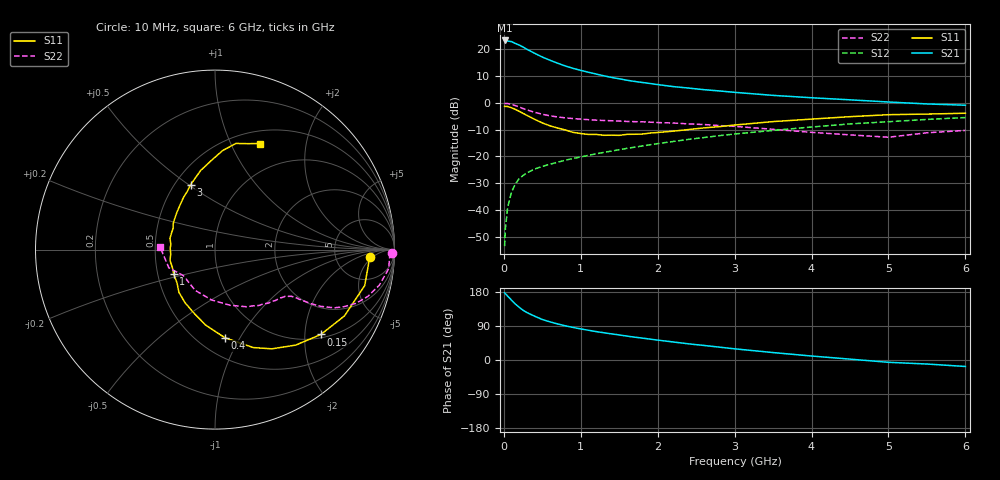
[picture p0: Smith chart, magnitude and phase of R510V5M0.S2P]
! SIEMENS Small Signal Semiconductors
! BFR183
! Si NPN RF Bipolar Junction Transistor in SOT23
! VCE = 10 V  IC = 5 mA
! Common Emitter S-Parameters:  May  1996
# GHz  S  MA  R  50
!  f  S11  S21  S12  S22
! GHz  MAG  ANG  MAG  ANG  MAG  ANG  MAG  ANG
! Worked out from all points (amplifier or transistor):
!   36 points, 10 MHz to 6 GHz, reference 50 ohm
!   highest |S21| = 23.4 dB at 10 MHz (marker M1)
!   |S21| within 3 dB of that: start of sweep to 282.1 MHz
!   unconditionally stable (mu >= 1): 1.095 GHz to 2.758 GHz
!   at 250 MHz: K = 0.41, MSG = 24.0 dB, |S12| = -27.1 dB
!   at 1.4 GHz: K = 1.05, MAG = 12.4 dB, |S12| = -18.0 dB
!   at 6 GHz: K = 0.87, MSG = 2.3 dB, |S12| = -5.5 dB
!   S11 on the Smith chart (normalised r, x): 10 MHz: 12, -4; 150 MHz: 1.09, -2.41; 400 MHz: 0.67, -0.87; 1 GHz: 0.61, -0.18; 3 GHz: 0.60, +0.51; 6 GHz: 0.64, +1.30
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0.01  0.8619 -2.9  14.71 177.5  0.0021 87.9  0.985 -1.2
0.02  0.8593 -5.3  14.47 174.9  0.0045 85.7  0.9738 -2.6
0.05  0.8579 -13.5  14.38 168.6  0.0112 81.7  0.9735 -6.3
0.1  0.8105 -27.1  13.98 157.9  0.0215 75.1  0.937 -12.2
0.15  0.7561 -38.7  12.91 147.6  0.0307 70.3  0.8898 -17.1
0.2  0.6967 -49.8  12.06 139.1  0.0384 66.0  0.8398 -20.9
0.25  0.6371 -60.2  11.07 131.3  0.044 62.5  0.7851 -23.9
0.3  0.5857 -68.7  10.06 125.2  0.0493 60.1  0.7398 -26.0
0.4  0.494 -83.6  8.467 115.6  0.0581 57.1  0.6692 -28.2
0.5  0.4232 -97.2  7.202 106.9  0.065 56.1  0.6138 -29.4
0.6  0.3726 -108.4  6.274 100.6  0.0715 56.0  0.5736 -30.0
0.7  0.3397 -119.4  5.522 95.1  0.078 56.2  0.5466 -30.5
0.8  0.3118 -130.1  4.9 90.2  0.0848 56.3  0.5249 -30.7
1  0.2678 -149.0  4.057 82.0  0.0976 57.3  0.4974 -31.5
1.1  0.2573 -158.0  3.742 78.5  0.1047 57.8  0.4863 -32.4
1.6  0.2588 165.9  2.656 63.0  0.1414 58.4  0.4505 -36.8
2.2  0.2964 135.9  2.021 47.6  0.1902 56.5  0.4212 -45.1
3  0.3861 110.7  1.577 29.5  0.2624 50.7  0.3646 -60.9
3.5  0.4478 100.3  1.383 19.6  0.3063 45.5  0.3212 -74.9
4.5  0.5532 85.6  1.142 2.3  0.4052 34.4  0.2527 -115.9
5.5  0.6185 72.6  0.957 -10.6  0.4914 22.5  0.2765 -158.5
6  0.6417 67.1  0.906 -17.1  0.5329 14.6  0.3064 177.3
